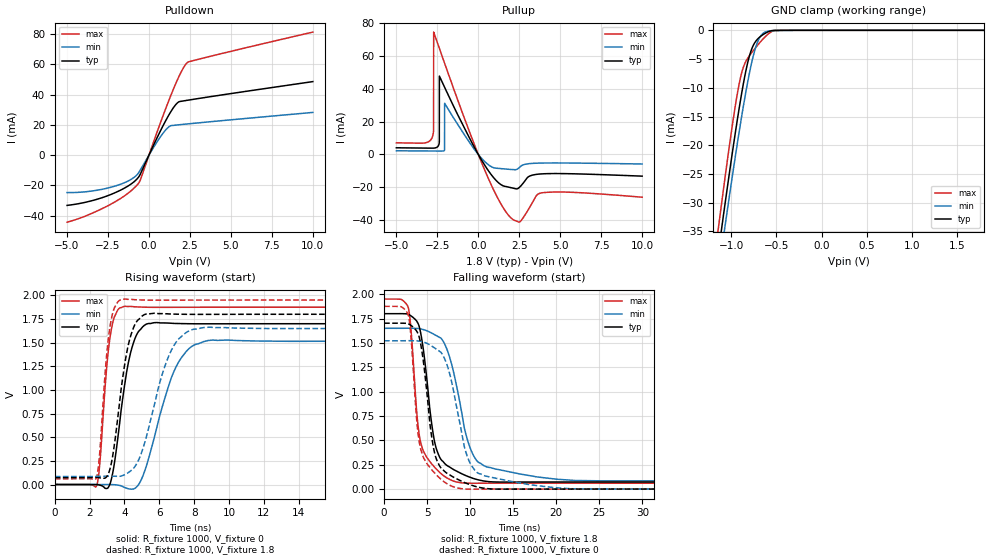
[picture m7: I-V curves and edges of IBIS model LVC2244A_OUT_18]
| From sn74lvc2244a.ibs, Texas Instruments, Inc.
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[Model]   LVC2244A_OUT_18
Model_type  3-state
Enable   Active-Low
Vref =   0
Rref =   1000
Cref =   30p
Vmeas =   0.9
| variable   typ   min   max
C_comp   7.15pF   6.80pF   7.52pF
| C_pullup   7.02pF   5.92pF   8.31pF
| C_pulldown   6.10pF   5.58pF   7.40pF
| C_tri-state   7.15pF   6.80pF   7.52pF
[Temperature Range]   40   100   -40
| Ambient temperature   25   85   -40
[Voltage range]   1.8   1.65   1.95
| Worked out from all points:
|   slope of the pulldown table from 0 to 0.27 V, typ, clamps not added: 42.5 ohm
|   slope of the pullup table from 0 to 0.27 V, typ, clamps not added: 58.8 ohm
|   GND clamp passes 1 mA (typ) near -0.67 V on its own axis
|   rising waveform, R_fixture 1000, V_fixture 0: 20-80 % time 797ps typ, 1.45ns min, 480ps max; typ from 0 V to 1.7 V
|   falling waveform, R_fixture 1000, V_fixture 1.8: 20-80 % time 1.53ns typ, 2.44ns min, 1.19ns max; typ from 1.8 V to 0.073 V
|   rising waveform, R_fixture 1000, V_fixture 1.8: 20-80 % time 777ps typ, 1.41ns min, 472ps max; typ from 0.073 V to 1.8 V
|   falling waveform, R_fixture 1000, V_fixture 0: 20-80 % time 1.47ns typ, 2.29ns min, 1.2ns max; typ from 1.7 V to 0 V
[GND Clamp]
| LVC2244A_OUT_18
|   Voltage   I(typ)   I(min)   I(max)
-5V       -524.6mA   -512.3mA   -544.5mA
-1.14V    -38.06mA   -41.69mA   -33.83mA
-1.115V   -35.19mA   -38.91mA   -30.82mA
-1.07V    -30.09mA   -33.97mA   -25.51mA
-955mV    -17.65mA   -21.77mA   -12.96mA
-885mV    -10.83mA   -14.84mA   -7.323mA
-830mV    -6.343mA   -9.869mA   -5.123mA
-775mV    -3.247mA   -5.592mA   -3.878mA
-715mV    -1.613mA   -2.237mA   -2.691mA
-650mV    -754uA     -537.1uA   -1.516mA
-515mV    -15.29uA   -57.67uA   -13.6uA
1.8V      35.25pA    10.02nA    -1.245nA
[Pulldown]
| LVC2244A_OUT_18
|   Voltage   I(typ)   I(min)   I(max)
-5V       -33.27mA   -24.8mA    -44.38mA
-3.6V     -30.49mA   -23.92mA   -39.06mA
-2.28V    -25.84mA   -21.13mA   -32.18mA
-1.235V   -20.15mA   -16.91mA   -24.86mA
-650mV    -14.75mA   -11.96mA   -18.81mA
-520mV    -12.37mA   -9.65mA    -16.25mA
480mV     11.17mA    8.561mA    14.81mA
1.11V     24.56mA    17.7mA     33.29mA
1.745V    34.65mA    19.97mA    50.03mA
2.1V      35.85mA    20.36mA    57.7mA
2.355V    36.3mA     20.63mA    61.37mA
10V       48.63mA    28.25mA    81.39mA
[Pullup]
| LVC2244A_OUT_18
|   Voltage   I(typ)   I(min)   I(max)
-5V       4.075mA    2.249mA    7.118mA
-2.795V   3.86mA     2.116mA    10.9mA
-2.73V    3.868mA    2.112mA    14.82mA
-2.725V   3.87mA     2.111mA    74.73mA
-2.385V   7.027mA    2.085mA    65.04mA
-2.38V    7.733mA    2.085mA    64.9mA
-2.375V   47.86mA    2.084mA    64.76mA
-2.06V    41.1mA     2.783mA    55.79mA
-2.055V   40.99mA    31.29mA    55.65mA
2.065V    -20.43mA   -9.209mA   -39.35mA
3.865V    -11.86mA   -5.245mA   -23.43mA
10V       -13.24mA   -5.813mA   -26.09mA
[Ramp]
| LVC2244A_OUT_18
| variable   typ   min   max
dV/dt_r   1.05/8.48E-10   0.94/1.56E-09   1.15/5.04E-10
dV/dt_f   1.04/1.60E-09   0.94/2.54E-09   1.13/1.21E-09
R_load = 1000
[Rising Waveform]
| LVC2244A_OUT_18
R_fixture =   1000
C_fixture =   0
L_fixture =   0
V_fixture =   0
V_fixture_min = 0
V_fixture_max = 0
|   Time   V(typ)   V(min)   V(max)
0s        640.8pV    3.394nV    28.48nV
2.41ns    -1.041mV   -482.9uV   -8.117mV
2.575ns   -6.182mV   -963.9uV   203.7mV
3.175ns   9.496mV    -202.5uV   1.561V
3.98ns    1.017V     -29.61mV   1.883V
4.51ns    1.496V     -48.38mV   1.88V
5.14ns    1.683V     132.6mV    1.874V
6.94ns    1.702V     1.237V     1.873V
8.785ns   1.698V     1.522V     1.874V
50ns      1.7V       1.515V     1.874V
[Falling Waveform]
| LVC2244A_OUT_18
R_fixture =   1000
C_fixture =   0
L_fixture =   0
V_fixture =   1.8
V_fixture_min = 1.65
V_fixture_max = 1.95
|   Time   V(typ)   V(min)   V(max)
0s        1.8V       1.65V      1.95V
2.83ns    1.792V     1.651V     1.857V
4.01ns    1.686V     1.647V     603.2mV
4.555ns   1.435V     1.637V     391.5mV
5.925ns   461.8mV    1.582V     219.2mV
7.84ns    212.9mV    1.282V     89.94mV
9.885ns   124.5mV    449.1mV    60.27mV
11.92ns   78.73mV    227.4mV    60.39mV
22.22ns   72.71mV    88.19mV    60.42mV
50ns      72.58mV    84.53mV    60.36mV
[Rising Waveform]
| LVC2244A_OUT_18
R_fixture =   1000
C_fixture =   0
L_fixture =   0
V_fixture =   1.8
V_fixture_min = 1.65
V_fixture_max = 1.95
|   Time   V(typ)   V(min)   V(max)
0s        72.55mV    84.43mV    60.35mV
2.375ns   74.63mV    85.34mV    67.16mV
2.55ns    71.58mV    86.02mV    274.7mV
3.155ns   156mV      88.44mV    1.655V
3.96ns    1.208V     99.62mV    1.959V
4.395ns   1.594V     150mV      1.957V
5.01ns    1.78V      353.6mV    1.95V
6.555ns   1.803V     1.365V     1.949V
7.965ns   1.798V     1.641V     1.949V
50ns      1.8V       1.65V      1.95V
[Falling Waveform]
| LVC2244A_OUT_18
R_fixture =   1000
C_fixture =   0
L_fixture =   0
V_fixture =   0
V_fixture_min = 0
V_fixture_max = 0
|   Time   V(typ)   V(min)   V(max)
0s        1.702V     1.522V     1.875V
2.83ns    1.695V     1.523V     1.779V
3.12ns    1.68V      1.523V     1.562V
3.95ns    1.592V     1.52V      567.6mV
4.55ns    1.318V     1.51V      328mV
5.86ns    373.6mV    1.449V     166.1mV
7.81ns    135.5mV    1.114V     31.96mV
9.665ns   55.52mV    334.3mV    -413.2uV
11.74ns   7.112mV    134.7mV    -27.03uV
50ns      28.95uV    98.73uV    10.68uV
